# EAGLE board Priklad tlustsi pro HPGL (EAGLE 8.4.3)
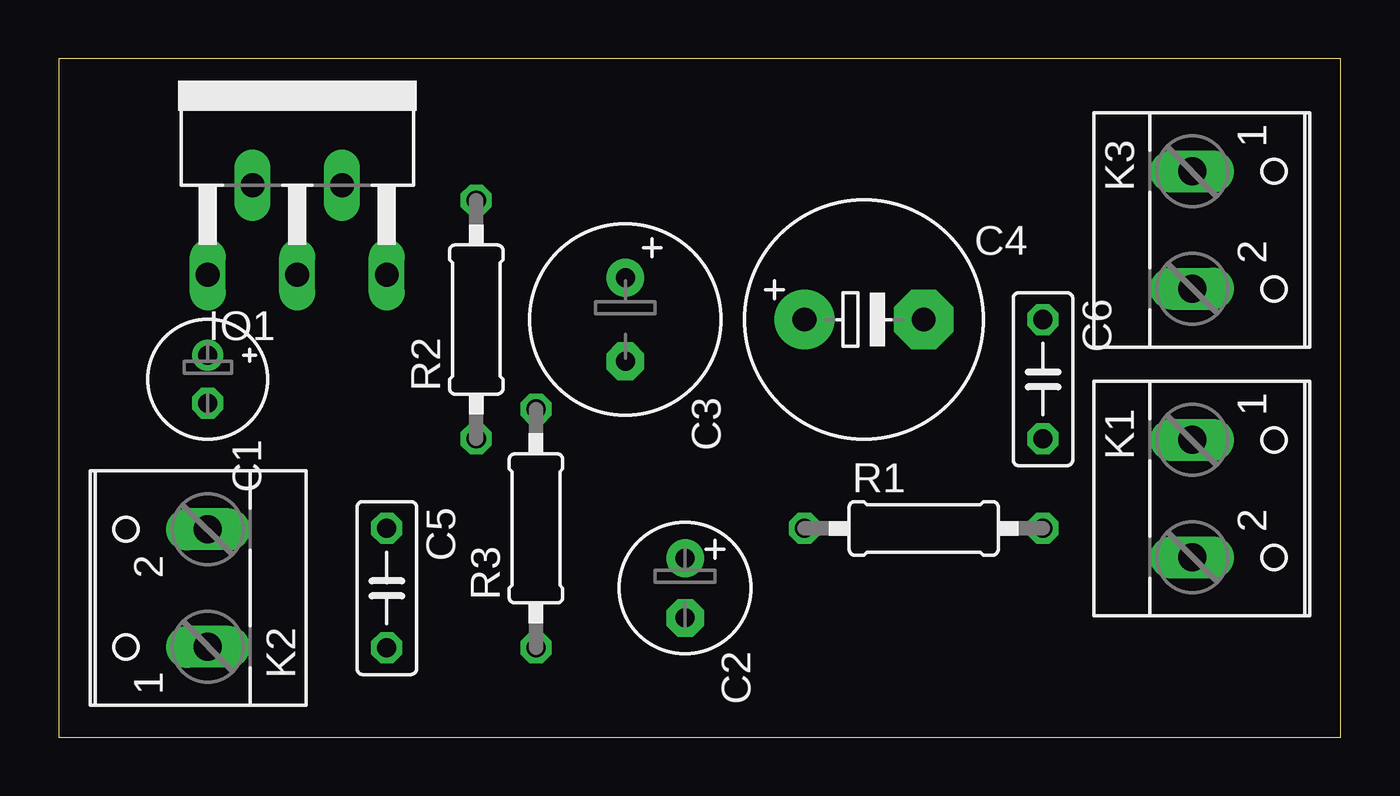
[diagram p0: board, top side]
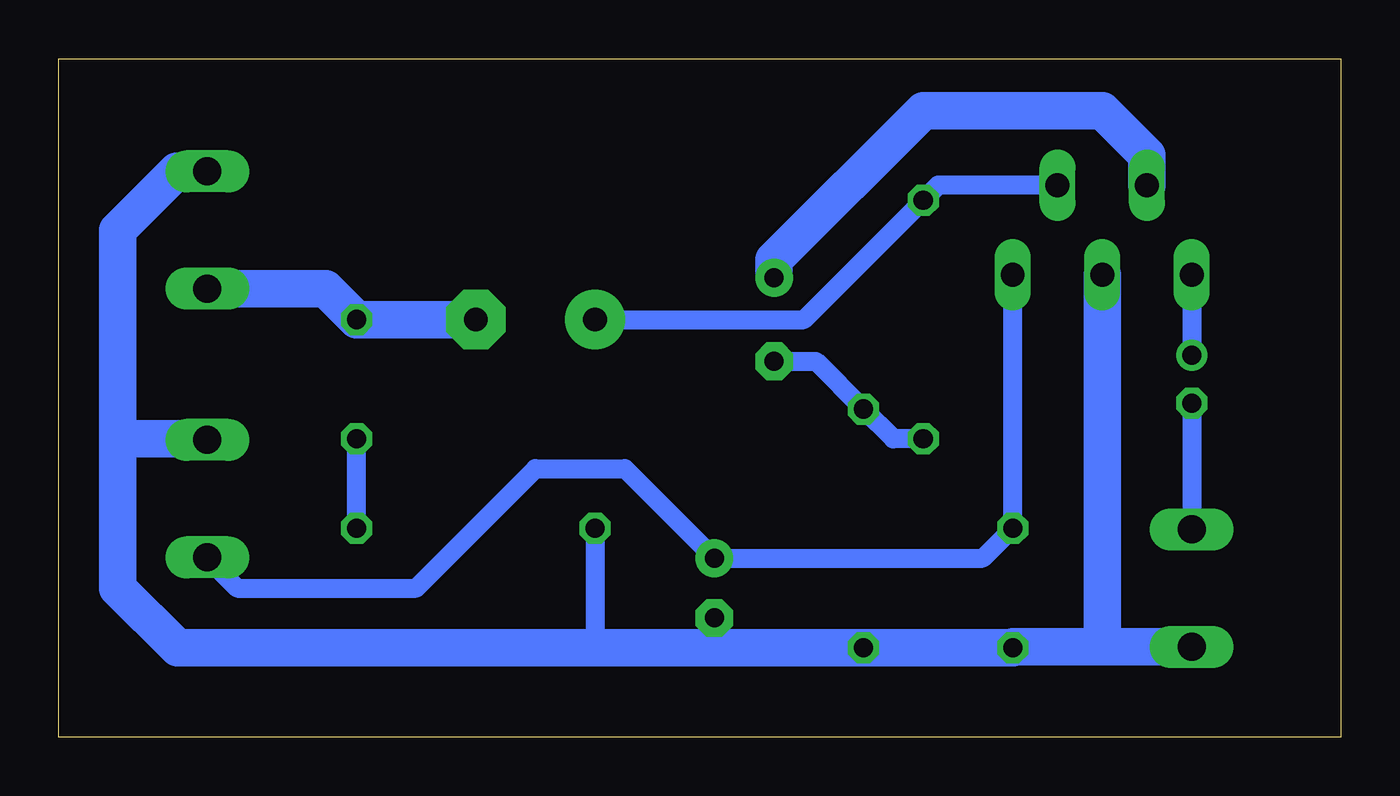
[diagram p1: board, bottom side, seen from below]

Size 54.59 x 28.88 mm. Coordinates in mm from the lower left corner, seen from the top.
Outline: 0,0 54.59,0 54.59,28.88 0,28.88 0,0
Copper layers (1*16): Top 0.035mm / dielectric 1.5mm / Bottom 0.035mm
Design rules "default": minimum track width 10mil, minimum drill 24mil, track to track 8mil, track to pad 8mil, pad to pad 8mil, via to via 8mil, smd to smd 8mil, copper to edge 40mil, drill to drill 8mil, minimum pad ring 10mil, minimum via ring 8mil, stop-mask expansion 4mil, vias tented up to drill 0mil, thermal gap 10mil

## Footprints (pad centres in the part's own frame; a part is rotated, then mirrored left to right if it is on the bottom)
E2-5 = drill 0.813 pad 1.27: + -1.016,0 | drill 0.813 pad 1.27 octagon: - 1.016,0
E2,5-6 = drill 0.813 pad 1.6: + -1.27,0 | drill 0.813 pad 1.6 octagon: - 1.27,0
E3,5-8 = drill 0.813 pad 1.6: + -1.778,0 | drill 0.813 pad 1.6 octagon: - 1.778,0
E5-10,5 = drill 1.016 pad 2.54: + -2.54,0 | drill 1.016 pad 2.54 octagon: - 2.54,0
C050-025X075 = drill 0.813 octagon: 1 -2.54,0; 2 2.54,0
CB360 = drill 1.016 long: 1 -3.81,-8.255; 2 -1.905,-4.445; 3 0,-8.255; 4 1.905,-4.445; 5 3.81,-8.255
W237-102 = drill 1.194 long: 1 -2.5,-1.27; 2 2.5,-1.27
0207/10 = drill 0.813 octagon: 1 -5.08,0; 2 5.08,0

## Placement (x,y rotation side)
C1  [E2-5]  6.35,15.24 270 top
C2  [E2,5-6]  26.67,6.35 270 top
C3  [E3,5-8]  24.13,17.78 270 top
C4  [E5-10,5]  34.29,17.78 0 top
C5  [C050-025X075]  13.97,6.35 270 top
C6  [C050-025X075]  41.91,15.24 270 top
IO1  TDA2003V  [CB360]  10.16,27.94 0 top
K1  [W237-102]  49.53,10.16 270 top
K2  [W237-102]  5.08,6.35 90 top
K3  [W237-102]  49.53,21.59 270 top
R1  [0207/10]  36.83,8.89 0 top
R2  [0207/10]  17.78,17.78 90 top
R3  [0207/10]  20.32,8.89 90 top

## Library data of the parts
C1-C6 R1-R3 = rcl
IO1 = linear
K1-K3 = con-wago-500; MPN: 237-102; OC_FARNELL: unknown; OC_NEWARK: 70K9898

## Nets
+18V: C2.+ C5.1 IO1.5 K1.2
GND: C2.- C5.2 IO1.3 K1.1 K2.1 K3.1 R1.1 R3.1
N$2: C1.+ IO1.1
N$4: C4.+ IO1.4 R2.2
N$5: C3.- R2.1 R3.2
N$7: C6.2 R1.2
N$8: C3.+ IO1.2
VST: C1.- K2.2
VYST: C4.- C6.1 K3.2

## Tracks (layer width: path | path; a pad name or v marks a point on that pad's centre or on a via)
+18V
  Bottom 0.8: IO1.5 C5.1 15.24,7.62 C2.+ 30.48,11.43 34.29,11.43 39.37,6.35 46.99,6.35 48.26,7.62 K1.2
GND
  Bottom 0.8: 48.3,12.7 K1.1 | 13.93,3.85 C5.2 | C2.- 26.67,3.81 | R1.1 31.75,3.81
  Bottom 1.6: K3.1 49.57,24.09 52.07,21.59 52.07,12.7 | 52.07,12.7 48.3,12.7 | K2.1 10.16,3.85 | 10.16,3.85 13.93,3.85 | C5.2 R3.1 26.67,3.81 31.75,3.81 49.53,3.81 52.07,6.35 52.07,12.7 | IO1.3 10.16,3.85
N$2
  Bottom 0.8: IO1.1 C1.+
N$4
  Bottom 0.8: IO1.4 17.14,23.49 R2.2 22.86,17.78 C4.+
N$5
  Bottom 0.8: R2.1 19.05,12.7 R3.2 22.35,16 C3.-
N$7
  Bottom 0.8: R1.2 C6.2
N$8
  Bottom 1.6: C3.+ 24.13,20.32 17.78,26.67 10.16,26.67 8.26,24.77 IO1.2
VST
  Bottom 0.8: C1.- K2.2
VYST
  Bottom 1.6: K3.2 43.22,19.09 C6.1 C4.-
